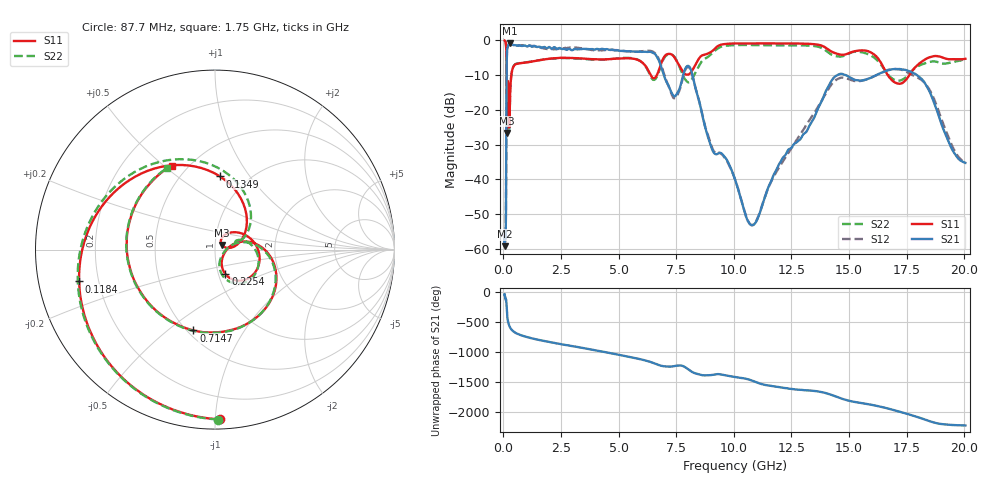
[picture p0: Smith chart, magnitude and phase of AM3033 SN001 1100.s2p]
# Hz S DB R 50
!freq MagS11 AngS11 MagS21 AngS21 MagS12 AngS12 MagS22 AngS22
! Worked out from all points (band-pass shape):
!   1601 points, 50 MHz to 20.05 GHz, reference 50 ohm
!   highest |S21| = -0.94 dB at 270.9 MHz (marker M1); lowest = -59.2 dB at 55.95 MHz (marker M2)
!   |S21| within 3 dB of the highest: 149.3 MHz to 6.572 GHz (6.423 GHz wide, 191 % of centre)
!   lowest |S11| = -26.7 dB at 151 MHz (marker M3), VSWR 1.10, Z = 54 + j2.75 ohm
!   |S11| at or under -10 dB: 137.6 MHz to 343.5 MHz (206 MHz wide, 85.6 % of centre); 6.383 GHz to 6.663 GHz (279.6 MHz wide, 4.29 % of centre); 16.68 GHz to 17.62 GHz (946.7 MHz wide, 5.52 % of centre)
!   |S22| runs from -26.0 to -0.1 dB; largest |S21 - S12| = 0.064
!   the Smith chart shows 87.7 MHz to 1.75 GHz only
!   S11 on the Smith chart (normalised r, x): 87.7 MHz: 0.06, -1.03; 118.4 MHz: 0.13, -0.11; 134.9 MHz: 0.75, +0.73; 225.4 MHz: 1.08, -0.30; 714.7 MHz: 0.54, -0.62; 1.75 GHz: 0.41, +0.53
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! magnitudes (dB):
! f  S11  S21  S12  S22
! 50 MHz  -0.1  -55.9  -58.6  -0.1
! 55.95 MHz  -0.2  -59.2  -56.8  -0.1
! 87.7 MHz  -0.5  -55.5  -56.0  -0.5
! 118.4 MHz  -2.2  -35.8  -35.8  -2.2
! 134.9 MHz  -7.8  -11.3  -11.3  -7.1
! 135.9 MHz  -8.6  -10.3  -10.3  -7.8
! 151 MHz  -26.7  -3.7  -3.7  -18.2
! 178.7 MHz  -12.3  -2.1  -2.1  -12.0
! 225.4 MHz  -16.5  -1.2  -1.2  -16.8
! 270.9 MHz  -19.8  -0.9  -0.9  -19.8
! 369.6 MHz  -8.9  -1.3  -1.3  -8.9
! 714.7 MHz  -6.6  -1.5  -1.5  -6.6
! 1.005 GHz  -6.4  -1.8  -1.5  -6.4
! 1.75 GHz  -5.6  -2.0  -2.4  -5.6
! 2.722 GHz  -5.1  -2.8  -2.4  -5.2
! 6.396 GHz  -10.2  -3.4  -3.1  -10.5
! 7.402 GHz  -4.8  -16.1  -16.7  -4.7
! 8.129 GHz  -9.3  -8.4  -8.6  -11.8
! 10.77 GHz  -1.0  -53.2  -53.1  -1.4
! 14.64 GHz  -4.2  -9.7  -10.8  -4.7
! 17.78 GHz  -8.5  -9.5  -10.1  -8.4
! 20.05 GHz  -5.4  -35.3  -35.1  -5.3
